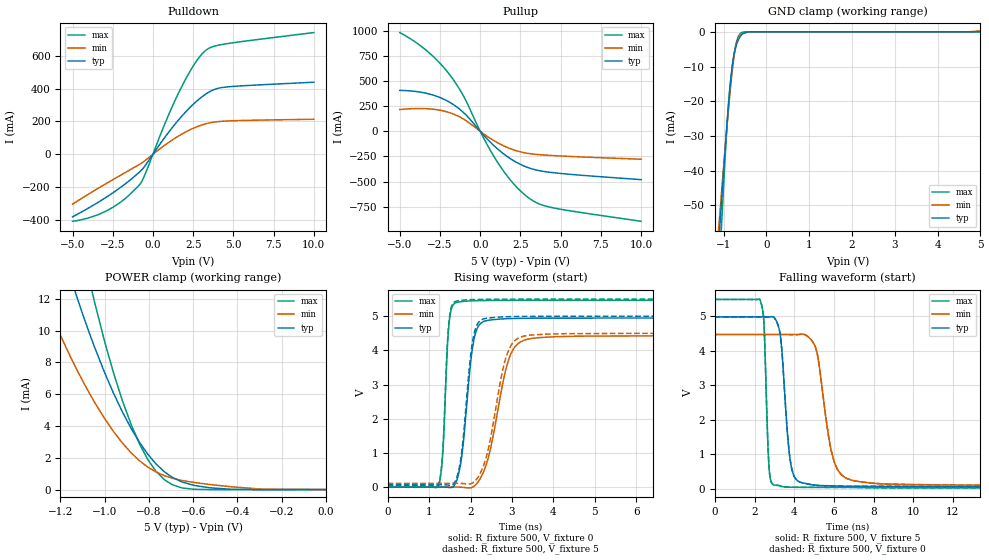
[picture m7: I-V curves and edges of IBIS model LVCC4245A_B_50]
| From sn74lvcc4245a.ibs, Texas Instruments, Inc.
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[Model]   LVCC4245A_B_50
Model_type  I/O
Vinl=1.65
Vinh=3.85
Enable   Active-Low
Vref =   0
Rref =   500
Cref =   50p
Vmeas =   2.5
| variable   typ   min   max
C_comp   11.0pF   NA   NA
| C_pullup   12.44pF   8.03pF   18.58pF
| C_pulldown   6.42pF   2.73pF   8.42pF
| C_tri-state   7.34pF   6.28pF   8.58pF
[Temperature Range]   40   100   -40
| Ambient temperature   25   85   -40
[Voltage range]   5   4.5   5.5
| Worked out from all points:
|   slope of the pulldown table from 0 to 0.75 V, typ, clamps not added: 7.17 ohm
|   slope of the pullup table from 0 to 0.75 V, typ, clamps not added: 5.88 ohm
|   GND clamp passes 1 mA (typ) near -0.59 V on its own axis
|   POWER clamp passes 1 mA (typ) near -0.72 V on its own axis
|   rising waveform, R_fixture 500, V_fixture 0: 20-80 % time 237ps typ, 440ps min, 119ps max; typ from 0 V to 4.95 V
|   falling waveform, R_fixture 500, V_fixture 5: 20-80 % time 375ps typ, 680ps min, 182ps max; typ from 4.98 V to 0.045 V
|   rising waveform, R_fixture 500, V_fixture 5: 20-80 % time 230ps typ, 413ps min, 118ps max; typ from 0.068 V to 5 V
|   falling waveform, R_fixture 500, V_fixture 0: 20-80 % time 375ps typ, 680ps min, 182ps max; typ from 4.98 V to 0.045 V
[GND Clamp]
| LVCC4245A_B_50
|   Voltage   I(typ)   I(min)   I(max)
-5V       -885.6mA   -763.3mA   -1.07A
-1.115V   -61.08mA   -56.77mA   -72.17mA
-1.075V   -53.76mA   -50.52mA   -62.48mA
-1.045V   -48.33mA   -45.88mA   -55.29mA
-920mV    -26.73mA   -27.26mA   -27.22mA
-880mV    -20.47mA   -21.7mA    -20.13mA
-835mV    -14.21mA   -15.85mA   -14.12mA
-775mV    -7.976mA   -9.104mA   -8.14mA
-705mV    -4.013mA   -3.724mA   -3.326mA
-650mV    -2.237mA   -1.708mA   -1.253mA
-570mV    -789.8uA   -645.8uA   -197uA
5V        22.96nA    282.9uA    618.8pA
[POWER Clamp]
| LVCC4245A_B_50
|   Voltage   I(typ)   I(min)   I(max)
-5V       437mA      297.9mA    722mA
-1.3V     20.38mA    13.01mA    30.09mA
-1.27V    18.83mA    11.97mA    27.57mA
-1.125V   12.08mA    7.52mA     16.71mA
-1.07V    9.868mA    6.08mA     13.22mA
-1.045V   8.93mA     5.473mA    11.75mA
-960mV    6.059mA    3.65mA     7.34mA
-880mV    3.838mA    2.306mA    4.076mA
-805mV    2.225mA    1.416mA    1.891mA
-730mV    1.119mA    876.3uA    619.5uA
-525mV    115.7uA    322.6uA    1.664uA
-84.45fV  22.96nA    29.73nA    1.104nA
[Pulldown]
| LVCC4245A_B_50
|   Voltage   I(typ)   I(min)   I(max)
-5V       -381.5mA   -303.9mA   -408.5mA
-3.8V     -315.9mA   -230.7mA   -381.6mA
-2.7V     -248.8mA   -166.7mA   -334.8mA
-1.75V    -182.7mA   -113.1mA   -271.7mA
-800mV    -105.3mA   -59.73mA   -181.7mA
-420mV    -60.16mA   -33mA      -105mA
905mV     125mA      67.11mA    224mA
1.665V    217.6mA    115.3mA    387.8mA
2.57V     310.3mA    160.8mA    547.7mA
3.29V     367.1mA    185.7mA    633.5mA
4.52V     409.2mA    202.1mA    672.4mA
10V       438.9mA    213.1mA    741.3mA
[Pullup]
| LVCC4245A_B_50
|   Voltage   I(typ)   I(min)   I(max)
-5V       407mA      216.8mA    982.6mA
-3.315V   376.7mA    224.5mA    800.5mA
-2.59V    341.4mA    211.9mA    691.9mA
-1.935V   291.9mA    186.6mA    570.5mA
-1.04V    186.5mA    122.1mA    350.9mA
155mV     -28.38mA   -18.82mA   -49.34mA
1.03V     -168.8mA   -109.8mA   -296.4mA
1.965V    -281.9mA   -178.6mA   -502.4mA
2.9V      -357.2mA   -218.2mA   -649.3mA
3.585V    -389.1mA   -231.5mA   -717.5mA
4.41V     -409.8mA   -240.7mA   -757.8mA
10V       -481.5mA   -278.2mA   -896.1mA
[Ramp]
| LVCC4245A_B_50
| variable   typ   min   max
dV/dt_r   2.98/2.44E-10   2.67/4.50E-10   3.29/1.21E-10
dV/dt_f   2.97/3.77E-10   2.65/6.83E-10   3.28/1.84E-10
R_load = 500
[Rising Waveform]
| LVCC4245A_B_50
R_fixture =   500
C_fixture =   0
L_fixture =   0
V_fixture =   0
V_fixture_min = 0
V_fixture_max = 0
|   Time   V(typ)   V(min)   V(max)
0s        1.657nV    80.35nV    186.3pV
1.225ns   384.8uV    85.95uV    48.51mV
1.33ns    150.9uV    247.1uV    1.007V
1.5ns     -15.1mV    859.1uV    4.983V
1.86ns    1.723V     -12.26mV   5.438V
2.03ns    3.925V     -10.75mV   5.45V
2.19ns    4.71V      165.6mV    5.456V
2.97ns    4.932V     3.887V     5.465V
3.7ns     4.944V     4.377V     5.466V
50ns      4.947V     4.428V     5.466V
[Falling Waveform]
| LVCC4245A_B_50
R_fixture =   500
C_fixture =   0
L_fixture =   0
V_fixture =   5
V_fixture_min = 4.5
V_fixture_max = 5.5
|   Time   V(typ)   V(min)   V(max)
0s        4.982V     4.471V     5.488V
2.285ns   4.982V     4.471V     5.458V
2.47ns    4.982V     4.471V     4.797V
2.755ns   4.98V      4.471V     441.6mV
3.38ns    3.96V      4.471V     65.19mV
4.01ns    342mV      4.47V      43.65mV
5.04ns    105.3mV    4.147V     41.16mV
5.985ns   84.03mV    839.1mV    40.82mV
7.12ns    72.28mV    222.4mV    37.01mV
50ns      44.9mV     70.66mV    27.18mV
[Rising Waveform]
| LVCC4245A_B_50
R_fixture =   500
C_fixture =   0
L_fixture =   0
V_fixture =   5
V_fixture_min = 4.5
V_fixture_max = 5.5
|   Time   V(typ)   V(min)   V(max)
0s        67.84mV    111.4mV    41.57mV
1.225ns   68.19mV    111.5mV    88.84mV
1.325ns   68.06mV    111.7mV    989mV
1.5ns     54.05mV    112.2mV    5.057V
1.82ns    1.394V     104.8mV    5.471V
2.015ns   3.981V     101.6mV    5.486V
2.175ns   4.788V     279.4mV    5.491V
2.895ns   4.986V     3.932V     5.498V
3.5ns     4.997V     4.453V     5.5V
50ns      5V         4.5V       5.5V
[Falling Waveform]
| LVCC4245A_B_50
R_fixture =   500
C_fixture =   0
L_fixture =   0
V_fixture =   0
V_fixture_min = 0
V_fixture_max = 0
|   Time   V(typ)   V(min)   V(max)
0s        4.982V     4.471V     5.488V
2.285ns   4.982V     4.471V     5.458V
2.47ns    4.982V     4.471V     4.797V
2.755ns   4.98V      4.471V     441.6mV
3.38ns    3.96V      4.471V     65.19mV
4.01ns    342mV      4.47V      43.65mV
5.04ns    105.3mV    4.147V     41.16mV
5.985ns   84.03mV    839.1mV    40.82mV
7.12ns    72.28mV    222.4mV    37.01mV
50ns      44.9mV     70.66mV    27.18mV
